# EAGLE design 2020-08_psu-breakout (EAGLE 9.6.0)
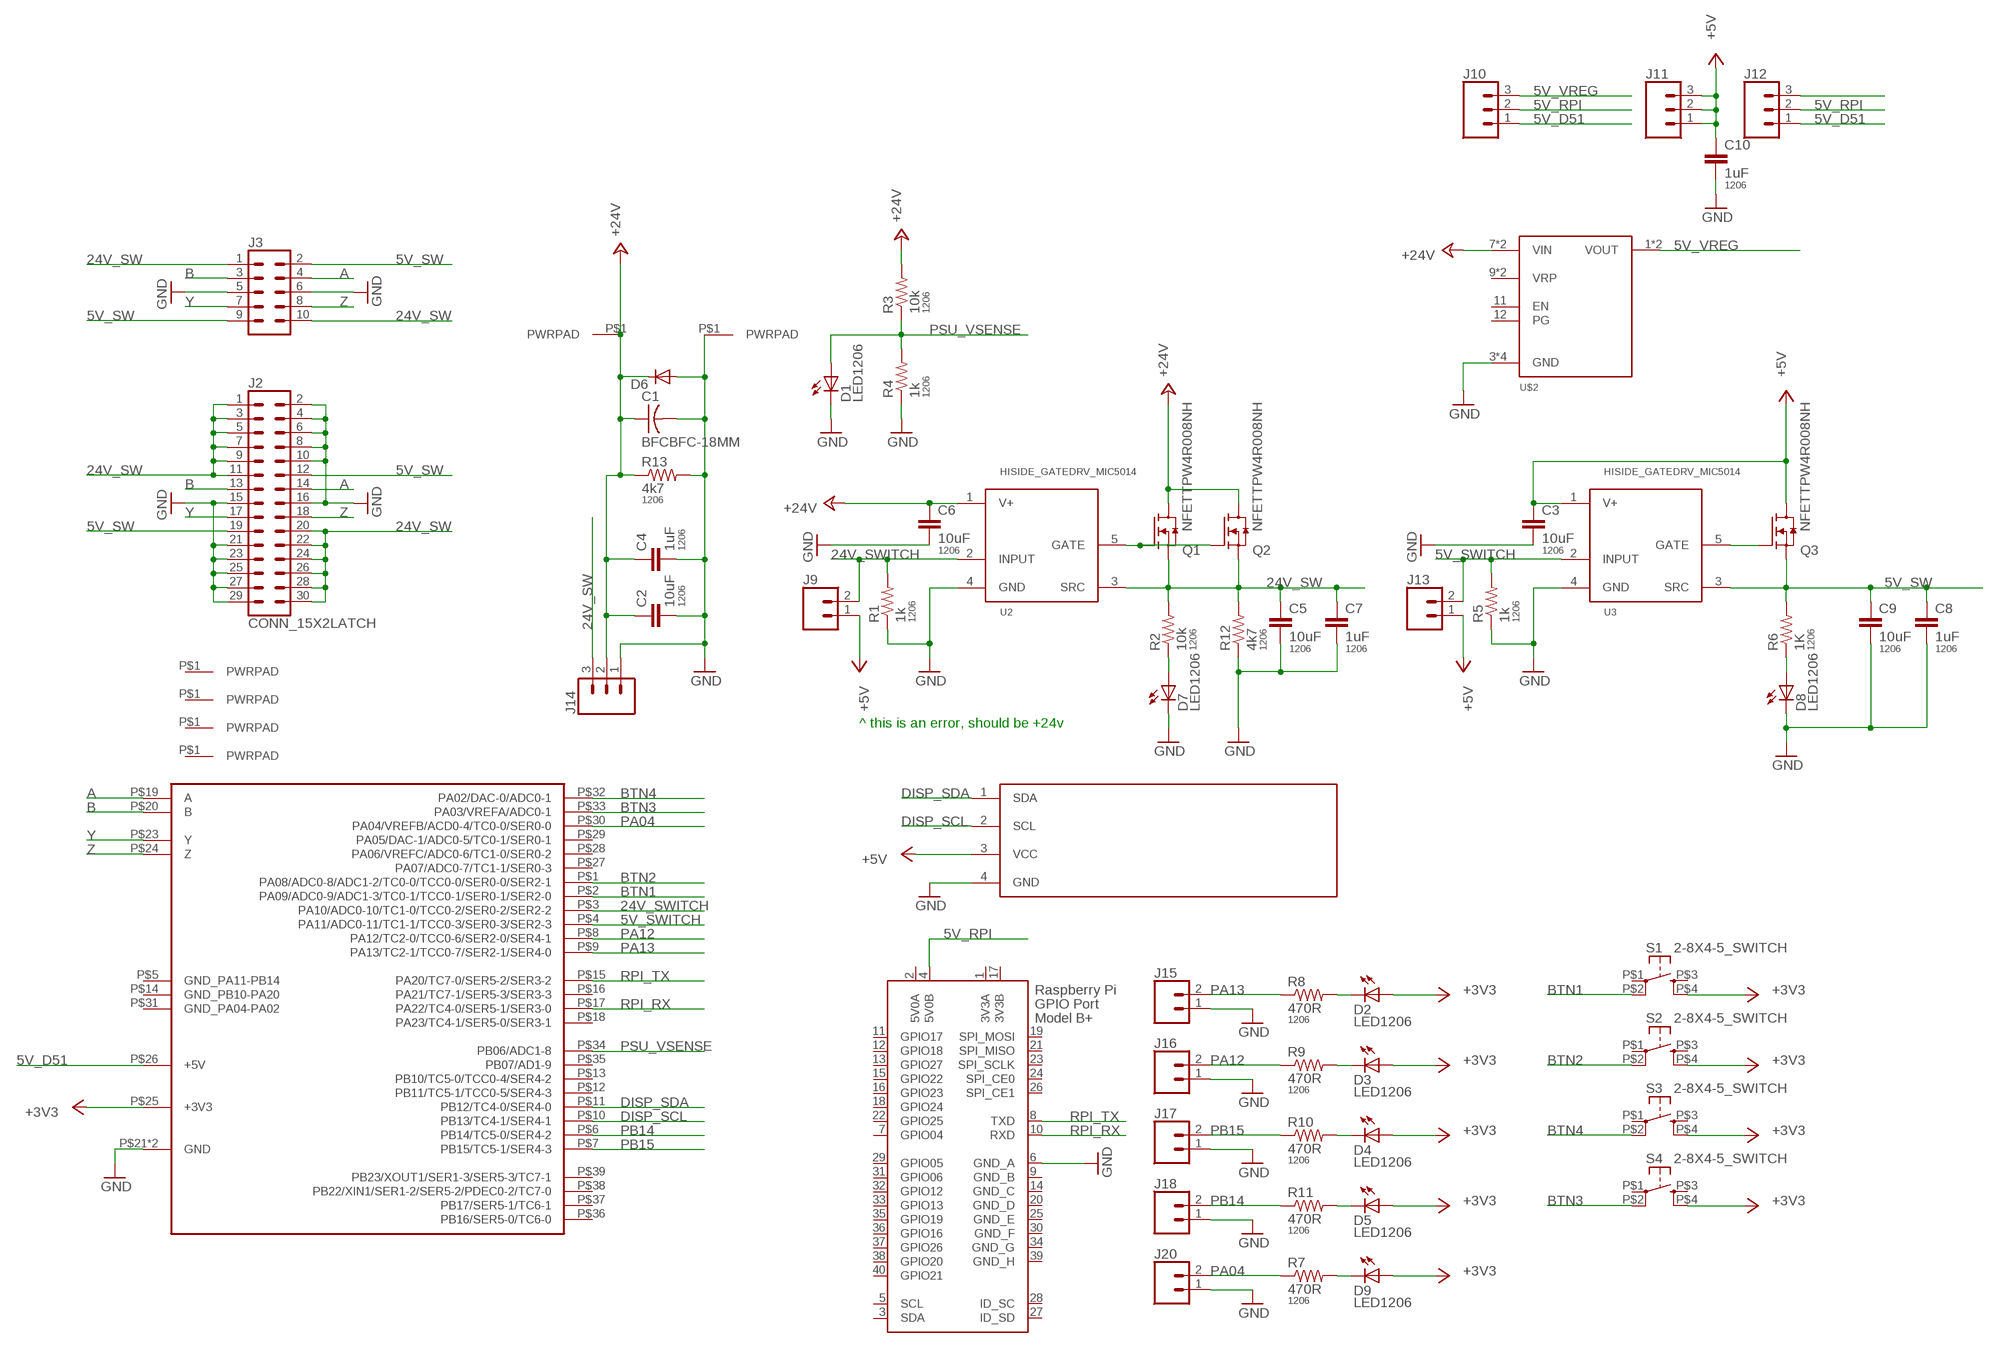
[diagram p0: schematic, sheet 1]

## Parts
C1  BFCBFC-18MM  [BFC-18MM-7-5MM]
C2  10uF  CAP1206  [1206]
C3  10uF  CAP1206  [1206]
C4  1uF  CAP1206  [1206]
C5  10uF  CAP1206  [1206]
C6  10uF  CAP1206  [1206]
C7  1uF  CAP1206  [1206]
C8  1uF  CAP1206  [1206]
C9  10uF  CAP1206  [1206]
C10  1uF  CAP1206  [1206]
D1  LED1206  [LED1206]
D2  LED1206  [LED1206]
D3  LED1206  [LED1206]
D4  LED1206  [LED1206]
D5  LED1206  [LED1206]
D6  DIODESMA403D  [SMA-403D]
D7  LED1206  [LED1206]
D8  LED1206  [LED1206]
D9  LED1206  [LED1206]
J1  I2C_OLED_MODULE  [I2C_MODULE_0.91INCH_PLANAR]
J2  CONN_15X2LATCH  [2X15-SHROUDED_LATCH]
J3  CONN_05X2SHD_LOCK_LATCH  [2X5-SHROUDED_LOCK_LATCH]
J4  PWRPADM3-SKINNY  [PWRPAD_3-25MM-SKINNY]
J5  PWRPADM3-SKINNY  [PWRPAD_3-25MM-SKINNY]
J6  PWRPADM3-SKINNY  [PWRPAD_3-25MM-SKINNY]
J7  PWRPADSOLDER  [SOLDER_ON]
J8  PWRPADSOLDER  [SOLDER_ON]
J9  CONN_02LOCK  [1X02_LOCK]
J10  CONN_03LOCK_NO_SILK  [1X03_LOCK_NO_SILK]
J11  CONN_03LOCK_NO_SILK  [1X03_LOCK_NO_SILK]
J12  CONN_03LOCK_NO_SILK  [1X03_LOCK_NO_SILK]
J13  CONN_02LOCK  [1X02_LOCK]
J14  CONN_03LOCK_NO_SILK  [1X03_LOCK_NO_SILK]
J15  CONN_02LOCK  [1X02_LOCK]
J16  CONN_02LOCK  [1X02_LOCK]
J17  CONN_02LOCK  [1X02_LOCK]
J18  CONN_02LOCK  [1X02_LOCK]
J19  PWRPADM3-SKINNY  [PWRPAD_3-25MM-SKINNY]
J20  CONN_02LOCK  [1X02_LOCK]
Q1  NFETTPW4R008NH  [DSOP-ADVANCE]
Q2  NFETTPW4R008NH  [DSOP-ADVANCE]
Q3  NFETTPW4R008NH  [DSOP-ADVANCE]
R1  1k  RESISTOR1206  [1206]
R2  10k  RESISTOR1206  [1206]
R3  10k  RESISTOR1206  [1206]
R4  1k  RESISTOR1206  [1206]
R5  1k  RESISTOR1206  [1206]
R6  1K  RESISTOR1206  [1206]
R7  470R  RESISTOR1206  [1206]
R8  470R  RESISTOR1206  [1206]
R9  470R  RESISTOR1206  [1206]
R10  470R  RESISTOR1206  [1206]
R11  470R  RESISTOR1206  [1206]
R12  4k7  RESISTOR1206  [1206]
R13  4k7  RESISTOR1206  [1206]
S1  2-8X4-5_SWITCH  [TACT-SWITCH-KMR6]
S2  2-8X4-5_SWITCH  [TACT-SWITCH-KMR6]
S3  2-8X4-5_SWITCH  [TACT-SWITCH-KMR6]
S4  2-8X4-5_SWITCH  [TACT-SWITCH-KMR6]
U1  UCBUS_MODULE_EXT  [UCBUS_MODULE_EXT]
U2  HISIDE_GATEDRV_MIC5014  [SOIC8_NOPAD]
U3  HISIDE_GATEDRV_MIC5014  [SOIC8_NOPAD]
U$2  POLOLU_D36VXXF6  [POLOLU_D36VXXF6]
X1  RASPI_BOARD_B+#_F  [RASPI_BOARD_B+_FULL]

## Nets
5V_D51: J10.1 J12.1 U1.P$26(+5V)
5V_RPI: J10.2 J12.2 X1.4(5V0B)
5V_SW: C8.1 C9.1 J2.12 J2.19 J3.2 J3.9 Q3.P$1(S) Q3.P$2(S) Q3.P$3(S) R6.2 U3.3(SRC)
5V_SWITCH: J13.2 R5.2 U1.P$4(PA11/ADC0-11/TC1-1/TCC0-3/SER0-3/SER2-3) U3.2(INPUT)
5V_VREG: J10.3 U$2.1(VOUT) U$2.2(VOUT)
24V_SW: C5.1 C7.1 J2.1 J2.3 J2.5 J2.7 J2.9 J2.11 J2.20 J2.22 J2.24 J2.26 J2.28 J2.30 J3.1 J3.10 J14.3 Q1.P$1(S) Q1.P$2(S) Q1.P$3(S) Q2.P$1(S) Q2.P$2(S) Q2.P$3(S) R2.2 R12.2 U2.3(SRC)
24V_SWITCH: J9.2 R1.2 U1.P$3(PA10/ADC0-10/TC1-0/TCC0-2/SER0-2/SER2-2) U2.2(INPUT)
+3V3: D2.1(A) D3.1(A) D4.1(A) D5.1(A) D9.1(A) S1.P$4(S1) S2.P$4(S1) S3.P$4(S1) S4.P$4(S1) U1.P$25(+3V3)
+5V: C3.1 C10.1 J1.3(VCC) J9.1 J11.1 J11.2 J11.3 J13.1 Q3.P$5(D) U3.1(V+)
+24V: C1.P$2 C2.1 C4.1 C6.1 D6.P$1(C) J7.P$1(PWRPAD) J14.2 Q1.P$5(D) Q2.P$5(D) R3.2 R13.1 U2.1(V+) U$2.7(VIN) U$2.8(VIN)
A: J2.14 J3.4 U1.P$19(A)
B: J2.13 J3.3 U1.P$20(B)
BTN1: S1.P$2(P1) U1.P$2(PA09/ADC0-9/ADC1-3/TC0-1/TCC0-1/SER0-1/SER2-0)
BTN2: S2.P$2(P1) U1.P$1(PA08/ADC0-8/ADC1-2/TC0-0/TCC0-0/SER0-0/SER2-1)
BTN3: S4.P$2(P1) U1.P$33(PA03/VREFA/ADC0-1)
BTN4: S3.P$2(P1) U1.P$32(PA02/DAC-0/ADC0-1)
DISP_SCL: J1.2(SCL) U1.P$10(PB13/TC4-1/SER4-1)
DISP_SDA: J1.1(SDA) U1.P$11(PB12/TC4-0/SER4-0)
GND: C1.P$1 C2.2 C3.2 C4.2 C5.2 C6.2 C7.2 C8.2 C9.2 C10.2 D1.2(C) D6.P$2(A) D7.2(C) D8.2(C) J1.4(GND) J2.2 J2.4 J2.6 J2.8 J2.10 J2.15 J2.16 J2.21 J2.23 J2.25 J2.27 J2.29 J3.5 J3.6 J8.P$1(PWRPAD) J14.1 J15.1 J16.1 J17.1 J18.1 J20.1 R1.1 R4.1 R5.1 R12.1 R13.2 U1.P$21(GND) U1.P$22(GND) U2.4(GND) U3.4(GND) U$2.3(GND) U$2.4(GND) U$2.5(GND) U$2.6(GND) X1.6(GND_A)
N$1: D3.2(C) R9.2
N$2: D7.1(A) R2.1
N$3: D2.2(C) R8.2
N$4: D4.2(C) R10.2
N$5: Q1.P$4(G) Q2.P$4(G) U2.5(GATE)
N$6: Q3.P$4(G) U3.5(GATE)
N$7: D8.1(A) R6.1
N$8: J12.3
N$9: D5.2(C) R11.2
N$10: D9.2(C) R7.2
PA04: J20.2 R7.1 U1.P$30(PA04/VREFB/ACD0-4/TC0-0/SER0-0)
PA12: J16.2 R9.1 U1.P$8(PA12/TC2-0/TCC0-6/SER2-0/SER4-1)
PA13: J15.2 R8.1 U1.P$9(PA13/TC2-1/TCC0-7/SER2-1/SER4-0)
PB14: J18.2 R11.1 U1.P$6(PB14/TC5-0/SER4-2)
PB15: J17.2 R10.1 U1.P$7(PB15/TC5-1/SER4-3)
PSU_VSENSE: D1.1(A) R3.1 R4.2 U1.P$34(PB06/ADC1-8)
RPI_RX: U1.P$17(PA22/TC4-0/SER5-1/SER3-0) X1.10(RXD)
RPI_TX: U1.P$15(PA20/TC7-0/SER5-2/SER3-2) X1.8(TXD)
Y: J2.17 J3.7 U1.P$23(Y)
Z: J2.18 J3.8 U1.P$24(Z)
Unconnected: J4.P$1(PWRPAD) J5.P$1(PWRPAD) J6.P$1(PWRPAD) J19.P$1(PWRPAD) S1.P$1(P) S1.P$3(S) S2.P$1(P) S2.P$3(S) S3.P$1(P) S3.P$3(S) S4.P$1(P) S4.P$3(S) U1.P$5(GND_PA11-PB14) U1.P$12(PB11/TC5-1/TCC0-5/SER4-3) U1.P$13(PB10/TC5-0/TCC0-4/SER4-2) U1.P$14(GND_PB10-PA20) U1.P$16(PA21/TC7-1/SER5-3/SER3-3) U1.P$18(PA23/TC4-1/SER5-0/SER3-1) U1.P$27(PA07/ADC0-7/TC1-1/SER0-3) U1.P$28(PA06/VREFC/ADC0-6/TC1-0/SER0-2) U1.P$29(PA05/DAC-1/ADC0-5/TC0-1/SER0-1) U1.P$31(GND_PA04-PA02) U1.P$35(PB07/AD1-9) U1.P$36(PB16/SER5-0/TC6-0) U1.P$37(PB17/SER5-1/TC6-1) U1.P$38(PB22/XIN1/SER1-2/SER5-2/PDEC0-2/TC7-0) U1.P$39(PB23/XOUT1/SER1-3/SER5-3/TC7-1) U$2.9(VRP) U$2.10(VRP) U$2.11(EN) U$2.12(PG) X1.3(SDA) X1.5(SCL) X1.7(GPIO04) X1.11(GPIO17) X1.12(GPIO18) X1.13(GPIO27) X1.15(GPIO22) X1.16(GPIO23) X1.18(GPIO24) X1.19(SPI_MOSI) X1.21(SPI_MISO) X1.22(GPIO25) X1.23(SPI_SCLK) X1.24(SPI_CE0) X1.26(SPI_CE1) X1.27(ID_SD) X1.28(ID_SC) X1.29(GPIO05) X1.31(GPIO06) X1.32(GPIO12) X1.33(GPIO13) X1.35(GPIO19) X1.36(GPIO16) X1.37(GPIO26) X1.38(GPIO20) X1.40(GPIO21)

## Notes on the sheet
- ^ this is an error, should be +24v

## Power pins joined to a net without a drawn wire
3V3A: X1.1(3V3A)
3V3B: X1.17(3V3B)
5V0A: X1.2(5V0A)
GND_B: X1.9(GND_B)
GND_C: X1.14(GND_C)
GND_D: X1.20(GND_D)
GND_E: X1.25(GND_E)
GND_F: X1.30(GND_F)
GND_G: X1.34(GND_G)
GND_H: X1.39(GND_H)

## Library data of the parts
C1 = power:BFC
C2-C10 = passives:CAP: Capacitor; PACKAGE: 1206
D1-D5 D7-D9 = lights:LED: LED
D6 = passives:DIODE: DIODE
J1 = lights:I2C_OLED_MODULE
J2 = SparkFun-Connectors:CONN_15X2
J3 = SparkFun-Connectors:CONN_05X2: Multi connection point. Often used as Generic Header-pin footprint for 0.1 inch spaced/style header connections For AVR SPI programming port, see special device with nice symbol: "AVR_SPI_PROG_5x2.dev" You can populate with any combo of single row headers, but if you'd like an exact match, check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
J4-J8 J19 = connector:PWRPAD
J9 J13 J15-J18 J20 = SparkFun-Connectors:CONN_02: Multi connection point. Often used as Generic Header-pin footprint for 0.1 inch spaced/style header connections
J10-J12 J14 = SparkFun-Connectors:CONN_03: Multi connection point. Often used as Generic Header-pin footprint for 0.1 inch spaced/style header connections On any of the 0.1 inch spaced packages, you can populate with these: Break Away Headers - Straight (PRT-00116) Break Away Male Headers - Right Angle (PRT-00553) Female Headers (PRT-00115)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
Q1-Q3 = power:NFET
R1-R13 = passives:RESISTOR: Resistor; PACKAGE: 1206
S1-S4 = passives:2-8X4-5_SWITCH
U1 = connector:UCBUS_MODULE_EXT
U2 U3 = power:HISIDE_GATEDRV_MIC5014
U$2 = power:POLOLU_D36VXXF6
X1 = raspberrypi_bastelstube_v13:RASPI_BOARD_B+#: Raspberry Pi GPIO connector with markings for the outer dimensions of the Raspberry Pi board model B+ with different sets of drill holes or mounting pads All pins connected

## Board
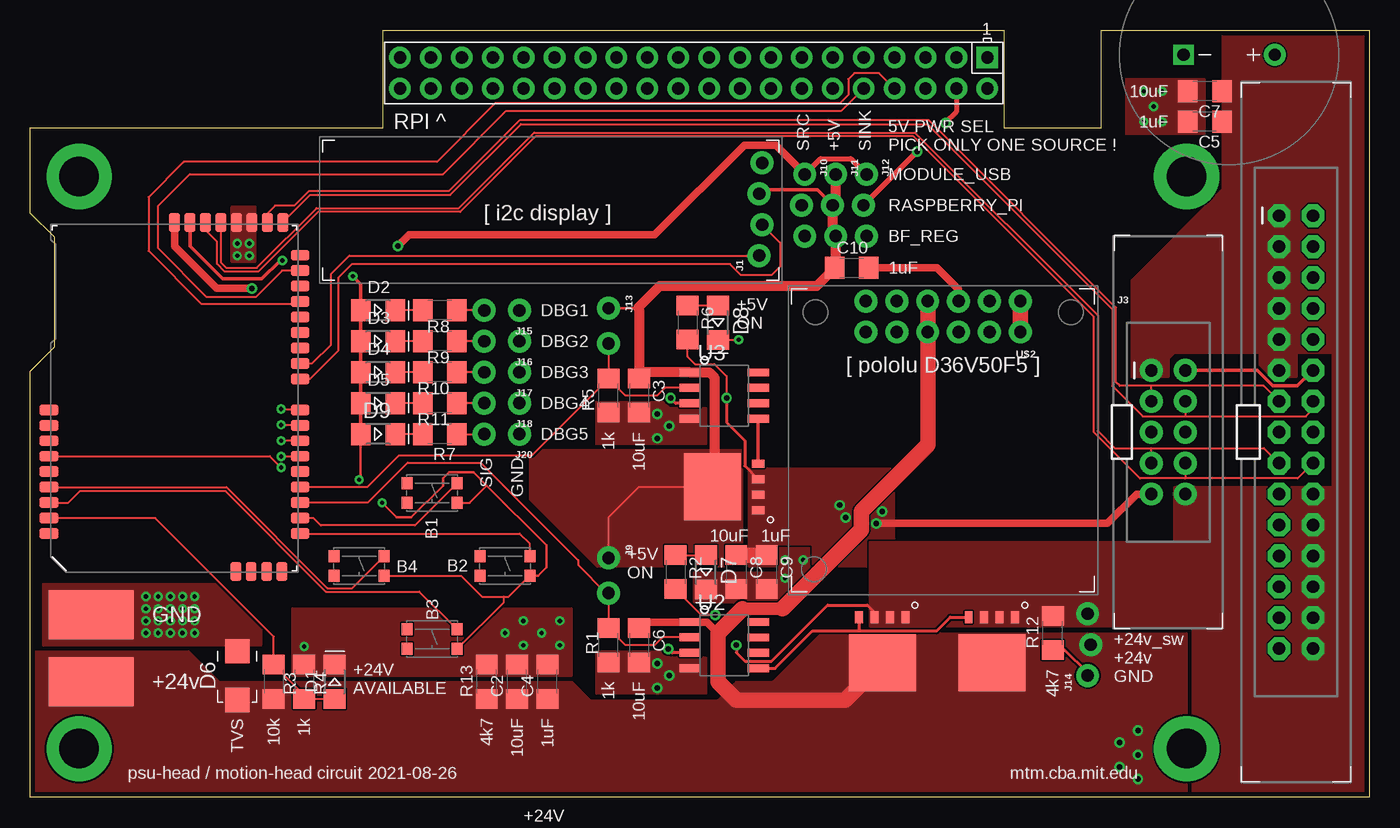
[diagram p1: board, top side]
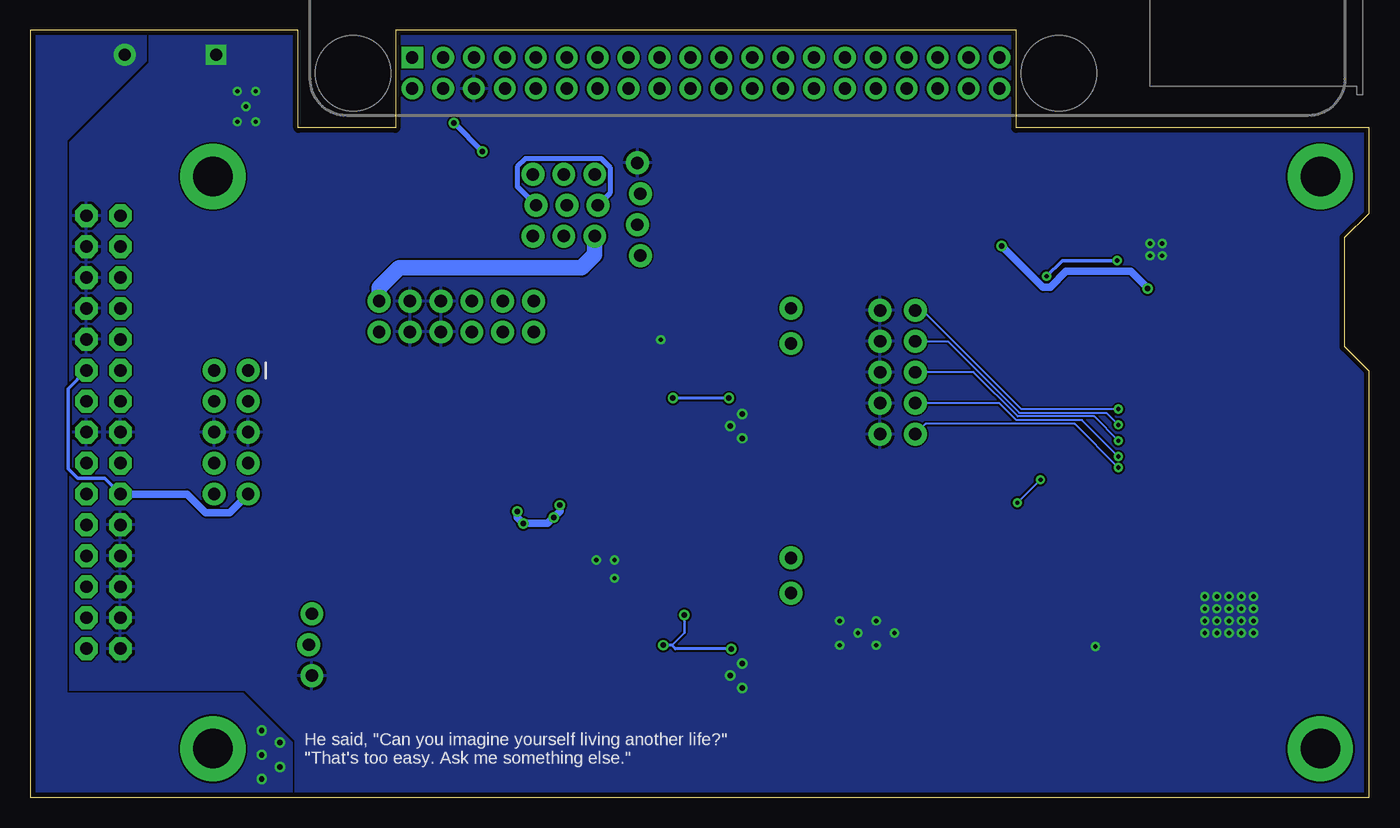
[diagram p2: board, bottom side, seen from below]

Size 110 x 63 mm. Coordinates in mm from the lower left corner, seen from the top.
Outline: 0,0 0,35 2,37 2,46 0,48 0,55 29,55 29,63 80,63 80,55 88,55 88,63 110,63 110,0 0,0
Copper layers (1*16): Top 0.035mm / dielectric 1.5mm / Bottom 0.035mm
Design rules "default *": minimum track width 6mil, minimum drill 0.35mm, track to track 6mil, track to pad 6mil, pad to pad 6mil, via to via 6mil, smd to smd 0mil, copper to edge 16mil, drill to drill 6mil, minimum pad ring 10mil, minimum via ring 8mil, stop-mask expansion 4mil, vias tented up to drill 35mil, thermal gap 10mil

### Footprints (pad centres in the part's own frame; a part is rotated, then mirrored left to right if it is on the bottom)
BFC-18MM-7-5MM = drill 1 pad 1.676 square: P$1 -3.75,0 | drill 1 pad 1.778: P$2 3.75,0
1206 = smd 1.6 x 1.8: 1 -1.4,0; 2 1.4,0
LED1206 = smd 1.6 x 1.803: 1 -1.422,0; 2 1.422,0
SMA-403D = smd 2 x 2: P$1 -2,0; P$2 2,0
I2C_MODULE_0.91INCH_PLANAR = drill 1.016 pad 1.88: 1 0,0.127; 2 2.54,-0.127; 3 5.08,0.127; 4 7.62,-0.127
2X15-SHROUDED_LATCH = drill 1.016 pad 1.88 octagon: 1 -1.397,17.78; 2 1.397,17.78; 3 -1.397,15.24; 4 1.397,15.24; 5 -1.397,12.7; 6 1.397,12.7; 7 -1.397,10.16; 8 1.397,10.16; 9 -1.397,7.62; 10 1.397,7.62; 11 -1.397,5.08; 12 1.397,5.08; 13 -1.397,2.54; 14 1.397,2.54; 15 -1.397,0; 16 1.397,0; 17 -1.397,-2.54; 18 1.397,-2.54; 19 -1.397,-5.08; 20 1.397,-5.08; 21 -1.397,-7.62; 22 1.397,-7.62; 23 -1.397,-10.16; 24 1.397,-10.16; 25 -1.397,-12.7; 26 1.397,-12.7; 27 -1.397,-15.24; 28 1.397,-15.24; 29 -1.397,-17.78; 30 1.397,-17.78
2X5-SHROUDED_LOCK_LATCH = drill 1.016 pad 1.88: 1 -1.397,5.08; 2 1.397,5.08; 3 -1.397,2.54; 4 1.397,2.54; 5 -1.397,0; 6 1.397,0; 7 -1.397,-2.54; 8 1.397,-2.54; 9 -1.397,-5.08; 10 1.397,-5.08
PWRPAD_3-25MM-SKINNY = drill 3.25 pad 5.35: P$1 0,0
SOLDER_ON = smd 4 x 7: P$1 0,0
1X02_LOCK = drill 1.016 pad 1.88: 1 -0.178,0; 2 2.718,0
1X03_LOCK_NO_SILK = drill 1.016 pad 1.88: 1 0,0.127; 2 2.54,-0.127; 3 5.08,0.127
DSOP-ADVANCE = smd 0.65 x 1: P$1 -1.905,-2.8; P$2 -0.635,-2.8; P$3 0.635,-2.8; P$4 1.905,-2.8 | smd 5.5 x 4.7: P$5 0,0.95
TACT-SWITCH-KMR6 = smd 0.9 x 1: P$1 -2.05,0.8; P$2 2.05,0.8; P$3 -2.05,-0.8; P$4 2.05,-0.8
UCBUS_MODULE_EXT = smd 0.889 x 1.524: P$1 3.175,-0.152; P$2 4.445,-0.152; P$3 5.715,-0.152; P$4 6.985,-0.152; P$5 8.255,-0.152; P$6 9.525,-0.152; P$7 10.795,-0.152; P$8 12.065,-0.152; P$9 13.335,-0.152; P$10 15.875,-0.152; P$11 17.145,-0.152; P$12 18.415,-0.152; P$13 19.685,-0.152; P$14 20.955,-0.152; P$15 22.225,-0.152; P$16 23.495,-0.152; P$17 24.765,-0.152; P$18 26.035,-0.152; P$27 13.335,20.472; P$28 12.065,20.472; P$29 10.795,20.472; P$30 9.525,20.472; P$31 8.255,20.472; P$32 6.985,20.472; P$33 5.715,20.472; P$34 4.445,20.472; P$35 3.175,20.472 | smd 1.524 x 0.889: P$19 28.727,1.27; P$20 28.727,2.54; P$21 28.727,3.81; P$22 28.727,5.08; P$23 28.727,6.35; P$24 28.727,7.62; P$25 28.727,8.89; P$26 28.727,10.16; P$36 0.05,1.32; P$37 0.05,2.59; P$38 0.05,3.86; P$39 0.05,5.13
SOIC8_NOPAD = smd 1.75 x 0.65: 1 -2.8,1.905; 2 -2.8,0.645; 3 -2.8,-0.625; 4 -2.8,-1.895; 5 2.8,-1.905; 6 2.8,-0.635; 7 2.8,0.635; 8 2.8,1.905
POLOLU_D36VXXF6 = drill 1.016 pad 1.88: 1 -6.35,-1.27; 2 -6.35,1.27; 3 -3.81,-1.27; 4 -3.81,1.27; 5 -1.27,-1.27; 6 -1.27,1.27; 7 1.27,-1.27; 8 1.27,1.27; 9 3.81,-1.27; 10 3.81,1.27; 11 6.35,-1.27; 12 6.35,1.27
RASPI_BOARD_B+_FULL = drill 1 pad 1.778 square: 1 8.37,51.23 | drill 1 pad 1.778: 2 8.37,53.77; 3 10.91,51.23; 4 10.91,53.77; 5 13.45,51.23; 6 13.45,53.77; 7 15.99,51.23; 8 15.99,53.77; 9 18.53,51.23; 10 18.53,53.77; 11 21.07,51.23; 12 21.07,53.77; 13 23.61,51.23; 14 23.61,53.77; 15 26.15,51.23; 16 26.15,53.77; 17 28.69,51.23; 18 28.69,53.77; 19 31.23,51.23; 20 31.23,53.77; 21 33.77,51.23; 22 33.77,53.77; 23 36.31,51.23; 24 36.31,53.77; 25 38.85,51.23; 26 38.85,53.77; 27 41.39,51.23; 28 41.39,53.77; 29 43.93,51.23; 30 43.93,53.77; 31 46.47,51.23; 32 46.47,53.77; 33 49.01,51.23; 34 49.01,53.77; 35 51.55,51.23; 36 51.55,53.77; 37 54.09,51.23; 38 54.09,53.77; 39 56.63,51.23; 40 56.63,53.77

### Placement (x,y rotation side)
C1  98.5,61 0 top
C2  40,9.5 90 top
C3  50,33 270 top
C4  42.5,9.5 90 top
C5  96.5,55.5 180 top
C6  50,12.5 270 top
C7  96.5,58 180 top
C8  58,18.5 270 top
C9  60.5,18.5 270 top
C10  67.5,43.5 0 top
D1  25,9.5 90 top
D2  28.57,40.01 0 top
D3  28.57,37.47 0 top
D4  28.57,34.92 0 top
D5  28.57,32.38 0 top
D6  17,10 90 top
D7  55.5,18.5 270 top
D8  56.5,39 270 top
D9  28.57,29.84 0 top
J1  60,44.5 90 top
J2  104,30 0 top
J3  93.5,30 0 top
J4  4,4 0 top
J5  95,51 0 top
J6  95,4 0 top
J7  5,9.5 270 top
J8  5,15 270 top
J9  47.5,19.5 270 top
J10  63.5,51.18 270 top
J11  66.04,51.18 270 top
J12  68.58,51.18 270 top
J13  47.5,40 270 top
J14  87,10 90 top
J15  40.01,40.01 180 top
J16  40.01,37.47 180 top
J17  40.01,34.92 180 top
J18  40.01,32.38 180 top
J19  4,51 0 top
J20  40.01,29.84 180 top
Q1  70,12 180 top
Q2  79,12 180 top
Q3  57,25.5 90 top
R1  47.5,12.5 90 top
R2  53,18.5 270 top
R3  20,9.5 270 top
R4  22.5,9.5 270 top
R5  47.5,33 90 top
R6  54,39 270 top
R7  33.66,29.84 180 top
R8  33.66,40.01 180 top
R9  33.66,37.47 180 top
R10  33.66,34.92 180 top
R11  33.66,32.38 180 top
R12  84,13.5 90 top
R13  37.5,9.5 90 top
S1  33,25 0 top
S2  39,19 0 top
S3  27,19 0 top
S4  33,13 0 top
U1  22,18.5 90 top
U2  57,12.5 0 top
U3  57,33 0 top
U$2  75,39.5 180 top
X1  87,112 180 top

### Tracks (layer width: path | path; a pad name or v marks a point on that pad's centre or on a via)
5V_D51  (via drill 0.45)
  Top 0.406: J10.1 64.92,52.48 67.41,52.48 J12.1
  Top 0.61: U1.P$26 11.84,45.26 15.29,41.81 v18.2,41.81 | v30.2,45.3 31.1,46.2 51.3,46.2 58.66,53.56 61.24,53.56 J10.1
  Bottom 0.61: v18.2,41.81 19.59,43.2 24.9,43.2 26.2,41.9 26.8,41.9 v30.2,45.3
5V_RPI  (via drill 0.45)
  Top 0.406: X1.4 76.09,56.29 v75.2,55.4 | v72.87,53.07 68.45,48.65 J12.2
  Bottom 0.406: J10.2 62.33,49.68 62.33,51.72 63.09,52.48 69.33,52.48 70,51.8 70,50.19 J12.2 | v75.2,55.4 v72.87,53.07
5V_SW  (via drill 0.45)
  Top 0.152: v57.2,32.8 57.2,34.6 56.2,35.6 54.6,35.6 54,36.2 R6.2
  Top 0.254: U3.3 53.02,32.38 v52.6,32.8 | v57.2,32.8 57.2,30.8 58.7,29.3 58.7,27.23 Q3.P$3
  Top 0.305: J3.2 100.82,35.08 102.1,33.8 104.12,33.8 J2.12
  Top 0.61: J3.9 90.92,24.92 88.5,22.5 v69.5,22.5
  Top 1.27: C8.1 C9.1
  Bottom 0.254: v52.6,32.8 v57.2,32.8
  Bottom 0.305: J2.12 106.9,33.58 106.9,27 106.1,26.2 103.88,26.2 J2.19
  Bottom 0.61: J2.19 97.12,24.92 95.6,23.4 93.62,23.4 J3.9 | v70,23.5 70,23 v69.5,22.5 67.5,22.5 v67,23 66.5,23.5 v66.5,24
  pour Top (rank 3, no thermals): 59,27 59,19 71,19 71,27
5V_SWITCH
  Top 0.152: U1.P$4 27.68,25.48 30.3,28.1 41.2,28.1 R5.2 | U3.2 52.15,33.65 51.5,33 48.9,33 R5.2 | J13.2 R5.2
5V_VREG
  Top 1.27: U$2.1 U$2.2
  Bottom 1.27: J10.3 63.63,44.57 64.7,43.5 79.7,43.5 81.35,41.85 U$2.1
24V_SW  (via drill 0.45)
  Top 0.203: R2.2 55.11,14.99 v56.27,14.99
  Top 0.254: U2.3 52.73,11.88 v52.4,12.2 | Q1.P$3 69.36,15.2 68.77,15.8 65.5,15.8 60.9,11.2 58.7,11.2 58,11.9 v58,12.5
  Bottom 0.203: v56.27,14.99 56.27,13.53 57.3,12.5
  Bottom 0.254: v52.4,12.2 57,12.2 57.3,12.5 v58,12.5
  pour Top (no thermals): 69,14 69,21 94,21 94,25.5 107,25.5 107,36.5 104,36.5 104,34.5 102,34.5 101,35.5 101,36.5 94,36.5 93.5,36 93.5,34.5 90.5,34.5 90.5,42.5 98,50 98,65 112,65 112,-2 95.5,-2 95.5,14
24V_SWITCH
  Top 0.152: U1.P$3 27.71,24.21 31,27.5 37,27.5 45,19.5 45,19.1 47.32,16.78 J9.2 R1.2 48.9,12.5 51.3,12.5 51.95,13.14 U2.2
+3V3  (via drill 0.35)
  Top 0.152: S1.P$4 36.1,24.2 37.5,25.6 | S3.P$4 35.4,18.2 37.1,16.5 38.9,16.5 | S2.P$4 41,18.2 39.3,16.5 38.9,16.5 | S4.P$4 38.9,16.05 38.9,16.5
  Top 0.203: v28.9,24.2 30.1,23 31.3,23 33.9,25.6 33.9,26.2 34.4,26.7 36.4,26.7 37.5,25.6 42.4,20.7 42.4,18.9 41.7,18.2 S2.P$4 | D9.1 27.15,26.25 v27,26.1
  Top 0.305: U1.P$25 13.11,45.29 15.8,42.6 19,42.6 20.5,44.1 v20.7,44.1 | v26.5,42.8 27.15,42.15 D2.1 D3.1 D4.1 D5.1 D9.1
  Bottom 0.203: v27,26.1 v28.9,24.2
  Bottom 0.305: v20.7,44.1 25.2,44.1 v26.5,42.8
+5V
  Top 0.152: J9.1 47.5,23 50,25.5 Q3.P$5
  Top 0.203: J13.1 49.92,40.18 50,40.1
  Top 0.305: J1.3 60.19,49.9 64.65,49.9 J11.2
  Top 0.61: 65.91,46.35 J11.3 | 50,40.3 50,40.1 | C3.1 50,34.8 50.1,34.91 | 56.2,25.65 Q3.P$5
  Top 0.813: J11.1 66.17,48.89 J11.2 65.91,46.35 | 50,40.3 51.7,42 64.6,42 C10.1 66.17,43.57 J11.3 | 50,40.1 50,34.8 | 50.1,34.91 U3.1 55.8,34.91 56.2,34.5 56.2,25.65
  pour Top (no thermals): 58.5,19 58.5,28.5 41,28.5 41,24.5 46.5,19
+24V  (via drill 0.45)
  Top 0.61: C6.1 50.51,14.4 U2.1 55.59,14.4 56.5,13.5
  Top 1.016: 58.5,15.5 61.8,15.5
  Top 1.27: U$2.7 U$2.8 73.73,28.95 68.28,23.5 68.28,21.98 61.8,15.5 | Q1.P$5 66.95,8 58,8 56.5,9.5 56.5,13.5 58.5,15.5
  other vias: 89.5,4.5 89.5,2.5 91,3.5 91,5.5 91,1.5
  pour Top (no thermals): -2,12 13,12 15.5,9.5 44.5,9.5 46,8 56.5,8 58,9.5 61,9.5 65,13.5 95,13.5 95,-2 -2,-2
  pour Bottom: 88.5,4.5 92.5,8.5 107,8.5 107,54 100.5,60.5 100.5,66 112.5,66 112.5,-3 88.5,-3
A
  Top 0.152: U1.P$19 23,49.5 34.5,49.5 40.3,55.3 73.7,55.3 88.9,40.1 88.9,33.8 91.4,31.3 94.9,31.3 | 94.9,31.3 104.8,31.3 105.4,31.9 J2.14 | J3.4 94.9,31.3
B
  Top 0.152: U1.P$20 19.46,47.96 20.1,48.6 21.67,48.6 22.88,49.8 34.37,49.8 40.17,55.6 73.83,55.6 89.2,40.23 89.2,34.1 89.5,33.8 92.1,33.8 | J2.13 101.34,33.8 92.1,33.8 | J3.3 92.1,33.8
BTN1
  Top 0.152: U1.P$2 23.25,22.95 23.85,22.34 31.59,22.34 S1.P$2
BTN2
  Top 0.152: S2.P$2 41.05,20.84 40.21,21.68 U1.P$1
BTN3
  Top 0.152: U1.P$33 3.12,24.21 4.08,25.18 15.99,25.18 24.27,16.89 31.95,16.89 S4.P$2
BTN4
  Top 0.152: U1.P$32 16.11,25.48 24.4,17.2 26.45,17.2 S3.P$2
DISP_SCL
  Top 0.152: J1.2 61.6,45.57 61.6,43.6 60.9,42.9 58.4,42.9 57.5,43.8 26.4,43.8 25.3,42.7 25.3,36.7 22.98,34.38 U1.P$10
DISP_SDA
  Top 0.152: U1.P$11 23.14,35.65 24.7,37.2 24.7,43 26.2,44.5 J1.1
GND  (via drill 0.35, 0.45)
  Top 0.152: D8.2 58.18,37.58 v58.2,37.6
  Top 0.254: R12.1 85,12.1 86.87,10.23 J14.1
  Top 0.61: C10.2 74.5,43.5 76.27,41.73 U$2.5
  other vias: 9.5,13.5 9.5,14.5 9.5,15.5 9.5,16.5 10.5,16.5 10.5,15.5 10.5,14.5 10.5,13.5 11.5,16.5 11.5,15.5 11.5,14.5 11.5,13.5 12.5,13.5 12.5,14.5 12.5,15.5 12.5,16.5 13.5,16.5 13.5,15.5 13.5,14.5 13.5,13.5 17,45.5 18,45.5 18,44.5 17,44.5 22.5,12.4 51.5,29.5 52.5,30.5 51.5,31.5 51.5,11 51.5,9 52.5,10 43.5,14.5 42,13.5 43.5,12.5 40.5,12.5 40.5,14.5 39,13.5 93,58 93,55.5 91.5,55.5 92.3,56.75 91.5,58 63.5,19.5 62,19.5 62,18
  pour Top (rank 2, no thermals): 1,12.5 19,12.5 19,17.5 1,17.5
  pour Top (rank 2, no thermals): 16.5,48.5 16.5,44 18.5,44 18.5,48.5
  pour Bottom (rank 2): -1,64 111,64 111,-1 -1,-1
  pour Top (no thermals): 46.5,32.5 52,32.5 52.5,32 55.5,32 55.5,29 46.5,29
  pour Top (no thermals): 46.5,12 52,12 52.5,11.5 55.5,11.5 55.5,8.5 46.5,8.5
  pour Top (no thermals): 44.5,10 44.5,15.5 21.5,15.5 21.5,10
  pour Top (rank 2, no thermals): 96.5,54.5 96.5,59 90,59 90,54.5
  pour Top (rank 2, no thermals): 64,16 64,20.5 61.5,20.5 61.5,18.5 54.5,18.5 54.5,16
N$1
  Top 0.152: R9.2 D3.2
N$2
  Top 0.152: R2.1 55.48,19.9 D7.1
N$3
  Top 0.152: R8.2 D2.2
N$4
  Top 0.152: R10.2 D4.2
N$5
  Top 0.254: U2.5 61.2,10.6 64.28,13.68 68.1,13.68 | Q2.P$4 75.59,14.8 74.47,13.68 68.1,13.68 | Q1.P$4 68.09,13.68 68.1,13.68
N$6
  Top 0.305: U3.5 Q3.P$4
N$7
  Top 0.152: R6.1 54.02,40.42 D8.1
N$9
  Top 0.152: R11.2 D5.2
N$10
  Top 0.152: R7.2 D9.2
PA04  (via drill 0.35)
  Top 0.152: U1.P$30 19.67,28.02 v20.6,27.09 | R7.1 J20.2
  Bottom 0.152: v20.6,27.09 24.19,30.68 36.45,30.68 J20.2
PA12  (via drill 0.35)
  Top 0.152: v20.6,30.6 22.12,30.6 U1.P$8 | J16.2 R9.1
  Bottom 0.152: J16.2 34.61,37.47 28.74,31.59 21.59,31.59 v20.6,30.6
PA13  (via drill 0.35)
  Top 0.152: U1.P$9 20.66,31.84 v20.6,31.9 | J15.2 R8.1
  Bottom 0.152: v20.6,31.9 28.58,31.9 36.69,40.01 J15.2
PB14  (via drill 0.35)
  Top 0.152: U1.P$6 22.13,28 v20.6,28 | J18.2 R11.1
  Bottom 0.152: v20.6,28 23.59,30.99 28.99,30.99 30.39,32.38 J18.2
PB15  (via drill 0.35)
  Top 0.152: U1.P$7 v20.61,29.3 v20.6,29.3 | J17.2 R10.1
  Bottom 0.152: v20.6,29.3 22.59,31.29 28.86,31.29 32.5,34.92 J17.2
PSU_VSENSE
  Top 0.152: U1.P$34 10.26,22.95 20,13.2 R3.1 22.5,8.4 R4.2 24.98,8.1 D1.1
RPI_RX
  Top 0.152: U1.P$17 20.66,43.27 18.5,41.1 14.5,41.1 10.5,45.1 10.5,48.6 13.1,51.2 33.9,51.2 39.1,56.4 66.64,56.4 X1.10
RPI_TX
  Top 0.152: X1.8 69.74,59.5 67.7,59.5 67.2,59 67.2,57.7 66.5,57 38.2,57 33.4,52.2 12.6,52.2 9.7,49.3 9.7,44.9 14.07,40.52 21.95,40.52 U1.P$15
Y
  Top 0.152: U1.P$23 15.65,43.95 16.1,43.5 18.6,43.5 23.5,48.4 35.2,48.4 41.4,54.6 72.7,54.6 87.7,39.6 87.7,30.1 89.1,28.7 92.1,28.7 | J2.17 101.36,28.7 92.1,28.7 | J3.7 92.1,28.7
Z
  Top 0.152: J2.18 104.14,26.2 94.9,26.2 | 94.9,26.2 91.17,26.2 87.39,29.97 87.39,39.47 72.57,54.3 41.53,54.3 35.33,48.09 23.63,48.09 18.73,43.2 15.97,43.2 15.35,43.82 15.35,45.66 14.38,46.62 U1.P$24 | J3.8 94.9,26.2

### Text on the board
tPlace: 10uF | RPI ^ | 1uF | 5V PWR SEL / PICK ONLY ONE SOURCE ! | SRC | +5V | SINK | MODULE_USB | RASPBERRY_PI | [ i2c display ] | BF_REG | 1uF | +5V / ON | DBG1 | DBG2 | [ pololu D36V50F5 ] | DBG3 | DBG4 | DBG5 | 1k | 10uF | SIG | GND | B1 | 10uF | 1uF | +5V / ON | B4 | B2 | GND | B3 | +24v_sw / +24v / GND | +24V / AVAILABLE | +24v | 1k | 10uF | 4k7 | TVS | 10k | 1k | 4k7 | 10uF | 1uF | psu-head / motion-head circuit 2021-08-26 | mtm.cba.mit.edu | +24V / ON
bPlace: He said, "Can you imagine yourself living another life?" / "That's too easy. Ask me something else."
